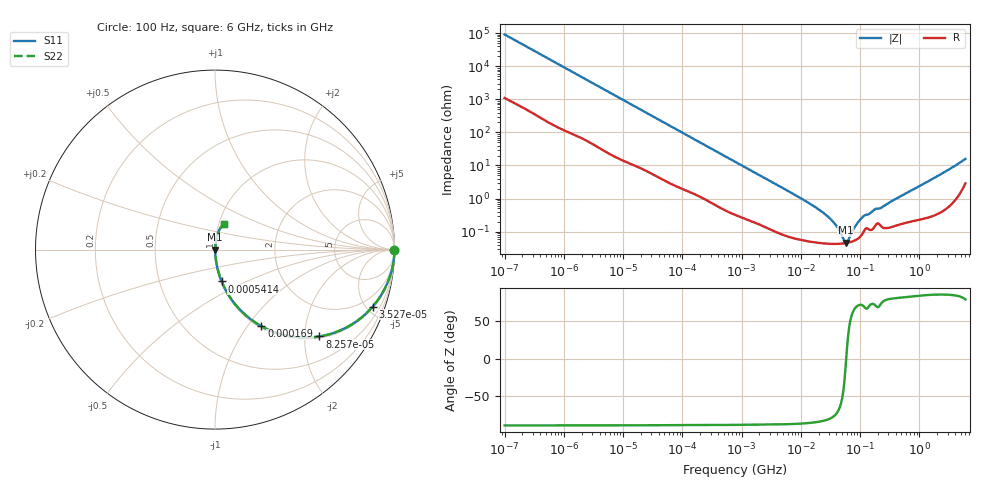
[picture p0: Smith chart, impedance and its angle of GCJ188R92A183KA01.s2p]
!Murata Part Number: GCJ188R92A183KA01
!These Parameters are Measured in Series Mode Connection
!Data Generated on Mar 13, 2026
!  o--ll--o
!Port1  Port2
!  o------o
!Operation Temp=25[degC], DC Bias Voltage=0[V]
!Freq. Start=100[Hz] Stop=6[GHz] 401[Steps]
# Hz S RI R 50
!Freq.(Hz) S11(Real) S11(Imag) S21(Real) S21(Imag) S12(Real) S12(Imag) S22(Real) S22(Imag)
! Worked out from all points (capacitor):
!   401 points, 100 Hz to 6 GHz, reference 50 ohm
!   read as one part in series: C = 17.2 nF near 109 Hz
!   lowest |Z| = 45.6 mohm at 56.99 MHz (marker M1)
!   series resonance near 58.37 MHz, so ESL is about 430 pH
!   S11 on the Smith chart (normalised r, x): 100 Hz: open; 35.27 kHz: 1.10, -5.49; 82.57 kHz: 1.05, -2.37; 169 kHz: 1.03, -1.17; 541.4 kHz: 1.01, -0.37; 6 GHz: 1.06, +0.31
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100  1 -0.00109  1.42e-05 0.00109  1.42e-05 0.00109  1 -0.00109
2008  0.9992 -0.0213  0.000756 0.0213  0.000756 0.0213  0.9992 -0.0213
10527  0.9864 -0.1085  0.0136 0.1085  0.0136 0.1085  0.9864 -0.1085
35265  0.8786 -0.3179  0.1214 0.3179  0.1214 0.3179  0.8786 -0.3179
40335  0.8482 -0.3501  0.1518 0.3501  0.1518 0.3501  0.8482 -0.3501
82567  0.5818 -0.4838  0.4182 0.4838  0.4182 0.4838  0.5818 -0.4838
169018  0.2587 -0.427  0.7413 0.427  0.7413 0.427  0.2587 -0.427
289253  0.1113 -0.3032  0.8887 0.3032  0.8887 0.3032  0.1113 -0.3032
541393  0.037 -0.1776  0.963 0.1776  0.963 0.1776  0.037 -0.1776
774597  0.0196 -0.127  0.9804 0.127  0.9804 0.127  0.0196 -0.127
2481164  0.00307 -0.0411  0.9969 0.0411  0.9969 0.0411  0.00307 -0.0411
1.555665e7  0.000523 -0.00628  0.9995 0.00628  0.9995 0.00628  0.000523 -0.00628
3.330331e7  0.000428 -0.00215  0.9996 0.00215  0.9996 0.00215  0.000428 -0.00215
4.165952e7  0.000426 -0.00126  0.9996 0.00126  0.9996 0.00126  0.000426 -0.00126
5.211241e7  0.000438 -0.000416  0.9996 0.000416  0.9996 0.000416  0.000438 -0.000416
5.699437e7  0.000448 -8.68e-05  0.9996 8.68e-05  0.9996 8.68e-05  0.000448 -8.68e-05
6.233367e7  0.000461 0.000244  0.9995 -0.000244  0.9995 -0.000244  0.000461 0.000244
8.154455e7  0.000539 0.00128  0.9995 -0.00128  0.9995 -0.00128  0.000539 0.00128
1.115611e8  0.000909 0.00265  0.9991 -0.00265  0.9991 -0.00265  0.000909 0.00265
3.124326e8  0.00137 0.00742  0.9986 -0.00742  0.9986 -0.00742  0.00137 0.00742
1.95892e9  0.00535 0.0455  0.9946 -0.0455  0.9946 -0.0455  0.00535 0.0455
6e9  0.0499 0.1439  0.9501 -0.1439  0.9501 -0.1439  0.0499 0.1439
